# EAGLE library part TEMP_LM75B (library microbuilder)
LM75B I2C Temperature Sensor The I2C-based LM75B can measure temperature between -55 and 125°C in 0.125°C increments (11-bit resolution). Digikey: 568-4768-1-ND For a 1.8V compatible part, look at the following pin and SW compatible parts: DS75LV - Mouser: 700-DS75LVS, Digikey: (TSSOP8) DS75LVU+-ND (SOIC8) DS75LVS+-ND
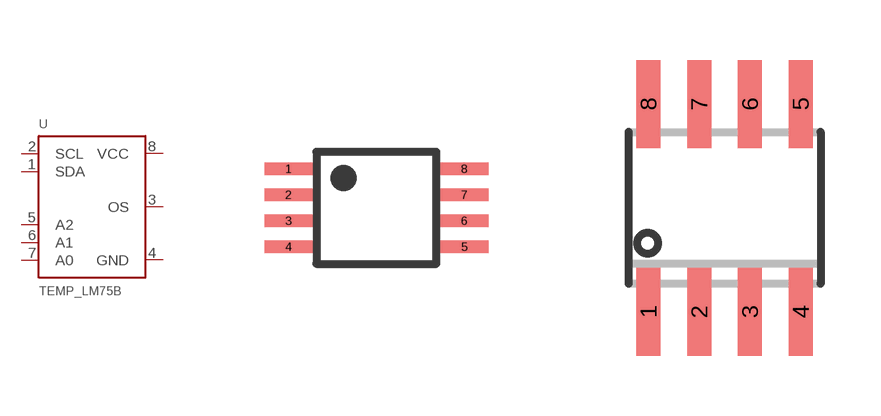
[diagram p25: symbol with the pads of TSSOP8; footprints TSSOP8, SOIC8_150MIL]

Designator prefix U

## TEMP_LM75B  [TSSOP8]
1  SDA
2  SCL
3  OS
4  GND  pwr
5  A2
6  A1
7  A0
8  VCC  pwr

## TEMP_LM75BSOIC  [SOIC8_150MIL]
Pads as for TSSOP8

## Footprint TSSOP8 (pad centres in mm)
Thin Shrink Small Outline Package 0.65mm Pitch, 3.0mm x 3.0mm
smd 1.2 x 0.305: 1 -2.2,0.975; 2 -2.2,0.325; 3 -2.2,-0.325; 4 -2.2,-0.975; 5 2.2,-0.975; 6 2.2,-0.325; 7 2.2,0.325; 8 2.2,0.975

## Footprint SOIC8_150MIL (pad centres in mm)
Small Outline IC - 150mil Wide
smd 0.6 x 2.2: 1 -1.905,-2.6; 2 -0.635,-2.6; 3 0.635,-2.6; 4 1.905,-2.6; 5 1.905,2.6; 6 0.635,2.6; 7 -0.635,2.6; 8 -1.905,2.6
